(* Logix 5000 AddOnInstructionDefinition export Gate_Slide; software revision 20.01 *)

TYPE Gate_Slide_Type :   // Slide Gate data
STRUCT
   Run_Status : BOOL;   // Run Status (1=running)
   Open_Status : BOOL;   // Open LS status (1=open gate)
   Close_Status : BOOL;   // Close LS status (1=closed gate)
   Any_Fail : BOOL;   // Overall Failure Alarm (1= alarm)
   Aux_Fail : BOOL;   // Auxiliary failure alarm (1=alarm)
   OL_Fail : BOOL;   // Overload alarm (1=alarm)
   HOA_Fail : BOOL;   // HOA-switch-not-in-auto alarm (1-alarm)
   Seq_Open : BOOL;   // Gate open initiated from sequence
   Seq_Close : BOOL;   // Gate close initiated from sequence
END_STRUCT
END_TYPE

ADD_ON_INSTRUCTION Gate_Slide   (* revision 1.3 *)
// Slide gate control
// Revision note:
// Correct name of "Dev_Num" input parameters
VAR_INPUT
   Open_Aux : BOOL; {required}   // Open auxillary contact physical input
   Close_Aux : BOOL; {required}   // Close auxiliary contact physical input
   OL_Trip : BOOL; {required}   // Overload trip contact physical input
   HOA_Switch : BOOL; {required}   // Hand-Off-Auto switch contact physical input (on when in Auto position)
   Open_LS : BOOL; {required}   // Gate-open limit switch physical input
   Close_LS : BOOL; {required}   // Gate-closed limit switch physical input
   Alarm_Reset : BOOL; {required}   // Resets alarms
   Maint : BOOL; {required}   // Unit Maintenance/Operate Privilege
   Man_Open : BOOL; {required}   // Manual open for unit
   Man_Close : BOOL; {required}   // Manual close for unit
   Select_Dev_Num : DINT; {required}   // Number of device started/stopped at OI
   This_Dev_Num : DINT; {required}   // Number of this device for OI control
END_VAR
VAR_OUTPUT
   Start_Open : BOOL; {access Read Only, required}   // Open motor starter contact physical input
   Start_Close : BOOL; {access Read Only, required}   // Close motor starter contact physical input
END_VAR
VAR_IN_OUT
   Tag : Gate_Slide_Type; {required}   // Slide Gate Tag
END_VAR
VAR
   Open_Req : BOOL;   // Internal used for open logic
   Close_Req : BOOL;   // Internal used for close logic
   Fail_Tmr : TIMER := (PRE := 20000);   // Timer for aux-fail alarm
END_VAR

ROUTINE Logic   (* ladder *)
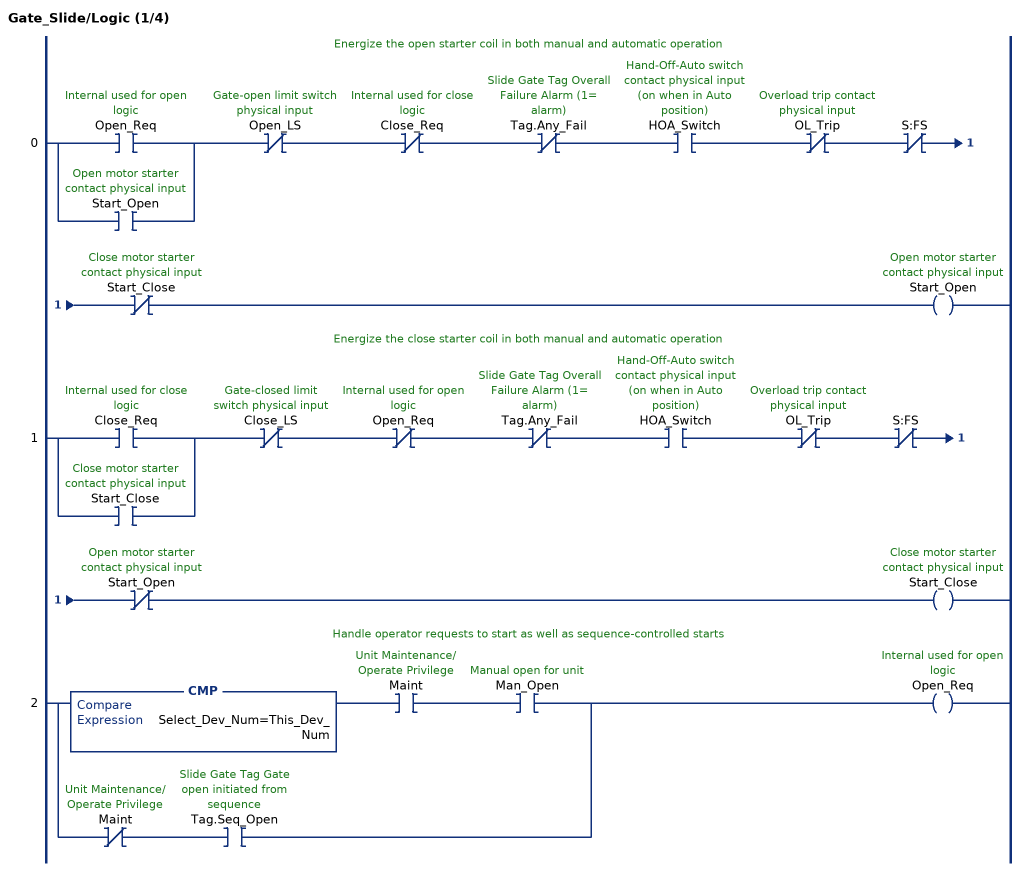
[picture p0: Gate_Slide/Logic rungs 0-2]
   // Energize the open starter coil in both manual and automatic operation
   0: [XIC(Open_Req) ,XIC(Start_Open) ]XIO(Open_LS)XIO(Close_Req)XIO(Tag.Any_Fail)XIC(HOA_Switch)XIO(OL_Trip)XIO(S:FS)XIO(Start_Close)OTE(Start_Open);
   // Energize the close starter coil in both manual and automatic operation
   1: [XIC(Close_Req) ,XIC(Start_Close) ]XIO(Close_LS)XIO(Open_Req)XIO(Tag.Any_Fail)XIC(HOA_Switch)XIO(OL_Trip)XIO(S:FS)XIO(Start_Open)OTE(Start_Close);
   // Handle operator requests to start as well as sequence-controlled starts
   2: [CMP(Select_Dev_Num=This_Dev_Num) XIC(Maint) XIC(Man_Open) ,XIO(Maint) XIC(Tag.Seq_Open) ]OTE(Open_Req);
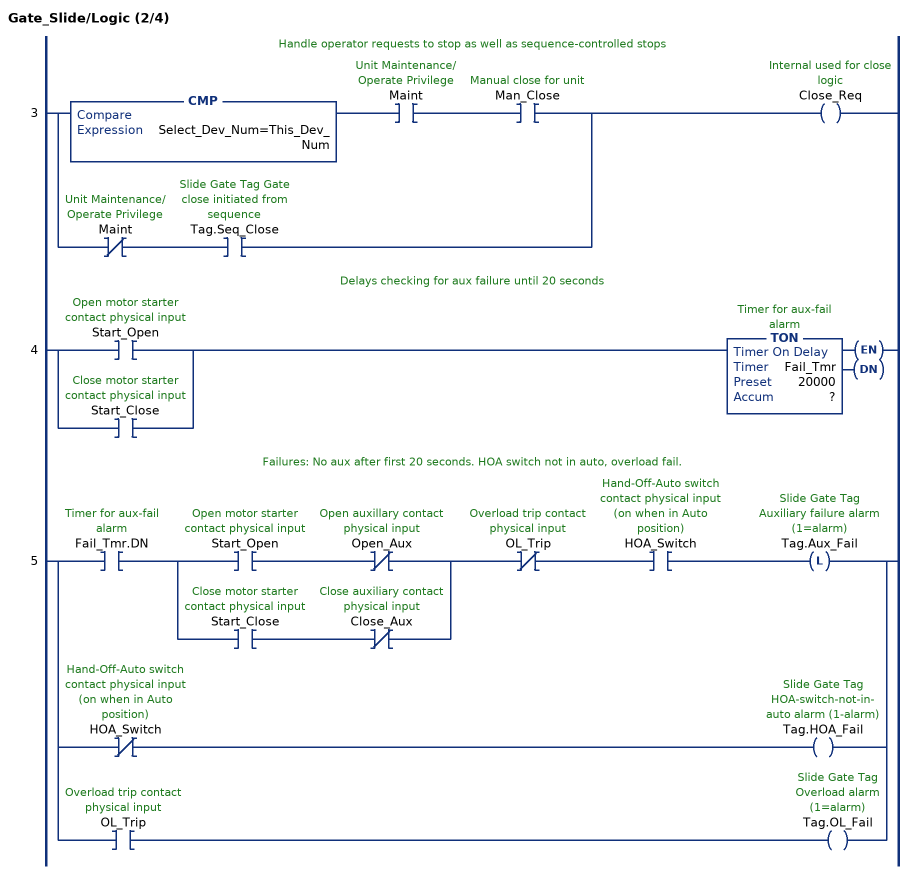
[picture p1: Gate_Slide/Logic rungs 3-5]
   // Handle operator requests to stop as well as sequence-controlled stops
   3: [CMP(Select_Dev_Num=This_Dev_Num) XIC(Maint) XIC(Man_Close) ,XIO(Maint) XIC(Tag.Seq_Close) ]OTE(Close_Req);
   // Delays checking for aux failure until 20 seconds
   4: [XIC(Start_Open) ,XIC(Start_Close) ]TON(Fail_Tmr,?,?);
   // Failures: No aux after first 20 seconds. HOA switch not in auto, overload fail.
   5: [XIC(Fail_Tmr.DN) [XIC(Start_Open) XIO(Open_Aux) ,XIC(Start_Close) XIO(Close_Aux) ] XIO(OL_Trip) XIC(HOA_Switch) OTL(Tag.Aux_Fail) ,XIO(HOA_Switch) OTE(Tag.HOA_Fail) ,XIC(OL_Trip) OTE(Tag.OL_Fail) ];
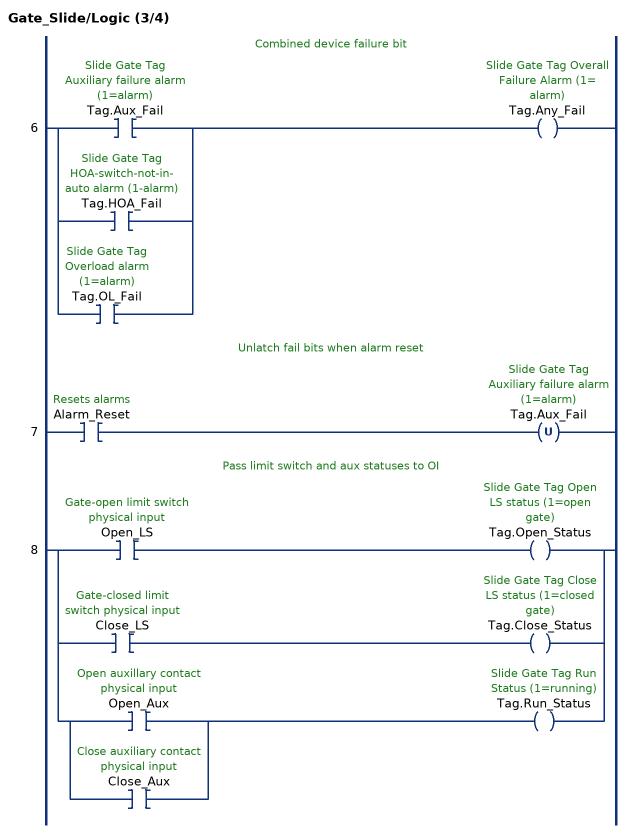
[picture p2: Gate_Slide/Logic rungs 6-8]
   // Combined device failure bit
   6: [XIC(Tag.Aux_Fail) ,XIC(Tag.HOA_Fail) ,XIC(Tag.OL_Fail) ]OTE(Tag.Any_Fail);
   // Unlatch fail bits when alarm reset
   7: XIC(Alarm_Reset)OTU(Tag.Aux_Fail);
   // Pass limit switch and aux statuses to OI
   8: [XIC(Open_LS) OTE(Tag.Open_Status) ,XIC(Close_LS) OTE(Tag.Close_Status) ,[XIC(Open_Aux) ,XIC(Close_Aux) ] OTE(Tag.Run_Status) ];
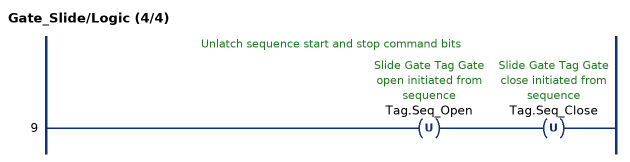
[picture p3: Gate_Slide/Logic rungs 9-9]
   // Unlatch sequence start and stop command bits
   9: OTU(Tag.Seq_Open)OTU(Tag.Seq_Close);
END_ROUTINE
END_ADD_ON_INSTRUCTION
